(* Logix 5000 Rung export; software revision 16.04 *)

MODULES
   Local : vendor None type None code None
   MVI56E_AFC : vendor None type None code None
END_MODULES

TYPE AFCEProveProcess :   // Prove process output from processor to the module
STRUCT
   Sequencing : AFCEProveSequencing;   // Prover sequencing
   Temperature : REAL;   // Temperature for Single Probe provers. And Inlet Temperature for Dual Probe Provers.
   OutletTemperature : REAL;   // Outlet Temperature for Provers with Dual Probes.
   SwitchBarTemperature : REAL;   // Switch bar temperature
   Pressure : REAL;   // Pressure for Single Probe provers. And Inlet Pressure for Dual Probe Provers.
   OutletPressure : REAL;   // Outlet Pressure for Provers with Dual Probes.
   ProverDensity : REAL;   // Prover density
END_STRUCT
END_TYPE

TYPE AFCEMeterControl :   // Enable/Disable Meter and Streams
STRUCT
   Meter : AFCEMeterControlMeter;   // Control the Meter
   Stream : AFCEMeterControlStream;   // Control the Meter Streams
   ResetAccumulators : AFCEMeterSignals;   // Resets for meter accumulators
END_STRUCT
END_TYPE

TYPE AFCEModbusMasterDataType :   // Modbus master data type
STRUCT
   Bit : BOOL;   // bit type
   Word : BOOL;   // word type (16-bit)
   Long : BOOL;   // long integer (32-bit)
   LongRemote : BOOL;   // long integer (32-bit)
END_STRUCT
END_TYPE

TYPE AFCEProveSequencing :   // AFC prove sequencing tag for phase selection and ball positioning
STRUCT
   Phase : AFCEProvePhaseBitmap;   // AFC phase sequencing
   BallPositionReady : BOOL;   // Ball position: Ready (Udir & Bdir only; fwd leg Bdir)
   BallPositionSealed : BOOL;   // Ball position: Sealed (Udir & Bdir only; fwd leg Bdir)
   BallPositionReadyBwdLeg : BOOL;   // Ball position: Ready bwd leg (Bdir only)
   BallPositionSealedBwdLeg : BOOL;   // Ball position: Sealed bwd leg (Bdir only)
END_STRUCT
END_TYPE

TYPE AFCEMeterDifferentialLiquid :   // Differential Liquid Meter
STRUCT
   Control : AFCEMeterControl;   // Meter Control
   Status : AFCEMeterStatus;   // Meter Status
   ProcessVariables : AFCEMeterDifferentialLiquidProcess;   // Input process variables to be transferred to the module
   Alarm : AFCEMeterDifferentialLiquidAlarm;   // Meter Alarms
   Archive : AFCEMeterDifferentialLiquidArchive;   // Archive
   Profile : AFCEMeterProfile;   // Module profile (meter type/product group) transfered from the module
   Calibration : AFCEMeterDifferentialLiqCal;   // Calibration
   BackPlaneReturn : AFCEMeterDifferentialLiqBackPlaneReturn;
END_STRUCT
END_TYPE

TYPE AFCEMeterDifferentialLiquidArchiveWrite :   // Write Archive
STRUCT
   Daily : BOOL;   // Set to 1 to write daily archive
   Hourly : BOOL;   // Set to 1 to write hourly archive
END_STRUCT
END_TYPE

TYPE AFCEUtil :   // Used for internal ladder logic usage. These values must not be changed by user application.
STRUCT
   Flags : AFCEFlag;   // Wallclock update commands
   CycleCounter : INT;   // Reflects current block ID calculated by ladder to be sent to the module
   Buffer : AFCEUtilBuffer;
   Block : AFCEUtilBlock;
END_STRUCT
END_TYPE

TYPE AFCEExtended :
STRUCT
   Trigger : BOOL;
   Data : AFCEExtendedData;
END_STRUCT
END_TYPE

TYPE AFCEModbusGatewayCommand :   // Modbus Gateway Command
STRUCT
   Config : AFCEModbusGatewayConfig;   // Config data to be entered by the user.
   Trigger : BOOL;   // Trigger the Command, when cleared module has responded.
   Data : INT[200];   // Contains modbus data written to the module (write commands)
END_STRUCT
END_TYPE

TYPE AFCEMeterDifferentialLiquidArchiveFetchT :   // Fetch Archive
STRUCT
   Trigger : BOOL;   // Trigger Archive Fetch
   Age : INT;   // 0 = Current Archive
   Error : AFCEMeterArchiveFetchError;   // Archive Fetch Error
   Default : AFCEMeterDifferentialLiquidArchiveDflt;   // Default Archive
   Raw : INT[100];   // Raw Archive
END_STRUCT
END_TYPE

TYPE AFCEMeterDifferentialLiqCal :   // Processor Mediated Calibration
STRUCT
   Request : AFCEMeterDifferentialLiqCalRequest;   // Calibration Request from module
   Response : AFCEMeterCalResponse;   // Processor Response
END_STRUCT
END_TYPE

TYPE AFCEMeterStatusStream :
STRUCT
   Active : INT;   // Current Active Stream
   Enabled : AFCEMeterStatusStreamEnabled;   // Enabled Streams
   Configured : AFCEMeterStatusStreamEnabled;   // Configured Streams
   EnableAlarm : AFCEMeterStatusStreamAlarm;   // Enable Alarms
END_STRUCT
END_TYPE

TYPE AFCEProveRunResults :   // Run results of the prove. Copied from the module to the pocessor
STRUCT
   CountAttempted : INT;   // Run count attempted
   CountCompleted : INT;   // Run count completed
   CountSelected : INT;   // Run count selected
   RunsSelected : INT;   // Bit Mapped Runs selected for calculations from completed runs
   NewMeterFactor : REAL;   // New meter factor
   ChangeInMeterFactor : REAL;   // Change in meter factor
END_STRUCT
END_TYPE

TYPE AFCEModbusMasterSwap :   // Modbus master swap words/ swap bytes
STRUCT
   SwapWords : BOOL;   // Swap words
   SwapBytes : BOOL;   // Swap bytes
END_STRUCT
END_TYPE

TYPE AFCEModbusMaster :   // Modbus Master. Port 3 must be configured as modbus master through AFC Manager to use this feature.
STRUCT
   Enable : BOOL;   // Enable the modbus master funcionality
   CommandIndex : INT;   // Selects which command index will be executed
   Command : AFCEModbusMasterCommand[10];   // Each command contains a specific modbus request to be sent out of the port
END_STRUCT
END_TYPE

TYPE AFCEMeterDifferentialLiqStandardDflt :   // Differential Liquid Meter Default Standard Data
STRUCT
   Meter_Alarms : DINT;   // Meter alarms
   NR_Acc_Net_Totalizer : DINT;   // Non-resettable accumulator, net, totalizer (m3)
   NR_Acc_Net_Residue : REAL;   // Non-resettable accumulator, net, residue (m3)
   FlowRate_Net : REAL;   // Flow rate, net (m3/h)
   NR_Acc_Gross_Totalizer : DINT;   // Non-resettable accumulator, gross, totalizer (m3)
   NR_Acc_GrossStandard_Totalizer : DINT;   // Non-resettable accumulator, gross standard, totalizer (m3)
   NR_Acc_Mass_Totalizer : DINT;   // Non-resettable accumulator, mass, totalizer (kg)
END_STRUCT
END_TYPE

TYPE AFCEFlag :   // Flags contains status information updated by ladder and also trigger bits for clock update
STRUCT
   AFCStopped : BOOL;   // Indicates that the module has sent a new input block to be processed by ladder - UPDATED BY LADDER
   AFCInputSequenceNum : INT;   // Meter number (0 -15) associated to blocks 1-16. Used to update "Profile" (meter type and product group.) UPDATED BY LADDER
END_STRUCT
END_TYPE

TYPE AFCEModbusPassThruBitData :   // AFC Modbus Pass-thru Bit Data
STRUCT
   Data : BOOL[2016];   // Contains received data for bit commands
END_STRUCT
END_TYPE

TYPE AFCEUtilBlockInterrupt :
STRUCT
   Now : BOOL;
   ModbusGateway : DINT;
   EnableDisable : BOOL;
   Analysis : DINT;
END_STRUCT
END_TYPE

TYPE AFCEFirmwareVersion :
STRUCT
   Major : SINT;   // Major Version number
   Minor : SINT;   // Minor Version number
   Revision : INT;   // Revision
END_STRUCT
END_TYPE

TYPE AFCEModbusGateway :   // Modbus Gateway
STRUCT
   Command : AFCEModbusGatewayCommand[10];   // Modbus gateway commands - contains setup and modbus data
END_STRUCT
END_TYPE

TYPE AFCEMeterDifferentialLiquidArchive :   // Different Liquid Archive
STRUCT
   Write : AFCEMeterDifferentialLiquidArchiveWrite;
   Fetch : AFCEMeterDifferentialLiquidArchiveFetch;
END_STRUCT
END_TYPE

TYPE AFCEMeterCalRequestActionType :
STRUCT
   ZeroShift : BOOL;   // Zero Shift
   SetZero : BOOL;   // Set Zero
   SetSpan : BOOL;   // Set Span
   SetMid1 : BOOL;   // Set Mid 1
   SetMid2 : BOOL;   // Set Mid 2
   SetMid3 : BOOL;   // Set Mid 3
END_STRUCT
END_TYPE

TYPE AFCEUtilBuffer :   // Buffer
STRUCT
   Input : INT[250];   // Input buffer contains the complete block to be copied from the module
   Output : INT[248];   // Output buffer contains data the complete block to be copied to the module
   Process : INT[240];
   ArchiveDay : INT[98];
   ArchiveHour : INT[98];
   Prove : INT[26];
   Analysis : INT[198];
   MeterEnableDisable : INT[4];
   StreamEnable : INT[48];
   StreamDisable : INT[48];
   StreamSelect : INT[32];
   MeterSignals : INT[32];
   Calibration : INT[36];
END_STRUCT
END_TYPE

TYPE AFCEUtilBlock :
STRUCT
   ProcessInput : INT;
   InterruptPending : AFCEUtilBlockInterrupt;
   InterruptComplete : AFCEUtilBlockInterrupt;
   NonInterruptPending : AFCEUtilBlockNonInterrupt;
   NonInterruptComplete : AFCEUtilBlockNonInterrupt;
END_STRUCT
END_TYPE

TYPE AFCEMeterSignals :   // Meter trigger accumulator and archive resets
STRUCT
   ResetAccumulator1 : BOOL;   // Set to 1 to reset resettable accumulator 1
   ResetAccumulator2 : BOOL;   // Set to 1 to reset resettable accumulator 2
   ResetAccumulator3 : BOOL;   // Set to 1 to reset resettable accumulator 3
   ResetAccumulator4 : BOOL;   // Set to 1 to reset resettable accumulator 4
END_STRUCT
END_TYPE

TYPE AFCEProve :   // Prove
STRUCT
   Process : AFCEProveProcess;   // Process Variables
   Signals : AFCEProveSignals;   // AFC Prove Signals (triggers the proving update)
   Config : AFCEProveConfig;   // AFC Prove Control (configuration settings)
   PulseCounts : AFCEProvePulseCount;   // Pulse counts to be updated at the end of the run/pass
   ConfigInput : AFCEProveInputConfig;   // AFC prover input configuration
   Status : AFCEProveStatus;   // AFC prover status
   ErrorCode : INT;   // Prove error code
   ProveControlsEcho : INT;   // AFC module Echos the state of the Prove Controls
   RequestedMeterEcho : INT;   // AFC module Echos the Meter number requested
   RequestedCurvePointEcho : INT;   // AFC module Echos the requested Curve Point
   RunResults : AFCEProveRunResults;   // Prove and run results
   ProveEnabled : BOOL;   // ON if prove is enabled. This flag is coped from inputbuffer[247]
END_STRUCT
END_TYPE

TYPE AFCEMeterControlStream :
STRUCT
   Selected : SINT;   // Stream to Enable or Disable and/or make active.
   EnableSelected : BOOL;   // Enable the Selected Stream
   DisableSelected : BOOL;   // Disable the Selected Stream
   SetSelectedToActive : BOOL;   // Set Selected to Active Stream
END_STRUCT
END_TYPE

TYPE AFCEProveConfig :   // Controls (configuration settings) associated to the prover
STRUCT
   Enable : AFCEProveConfigEnable;   // Controls at enable
   Accept : AFCEProveConfigAccept;   // Controls at accept
END_STRUCT
END_TYPE

TYPE AFCEWallclock :
STRUCT
   GetAFCTime : BOOL;   // Get current AFC Time
   SetAFCTimeFromPLCTime : BOOL;   // Set AFC time from PLC time. Updates current AFC time
   EnableLocalDateTime : BOOL;   // Enable Local Date Time.
   AFCTime : AFCETime;   // Coordinated Universal Time. Updated by either getting or setting AFC time.
END_STRUCT
END_TYPE

TYPE AFCEMeterCalRequestActionValue :
STRUCT
   ZeroShift : AFCEMeterCalRequestValue;   // Zero Shift
   SetZero : AFCEMeterCalRequestValue;   // Set Zero
   SetSpan : AFCEMeterCalRequestValue;   // Set Span
   SetMid1 : AFCEMeterCalRequestValue;   // Set Mid 1
   SetMid2 : AFCEMeterCalRequestValue;   // Set Mid 2
   SetMid3 : AFCEMeterCalRequestValue;   // Set Mid 3
END_STRUCT
END_TYPE

TYPE AFCEMeterStatus :   // Status
STRUCT
   Meter : AFCEMeterStatusMeter;   // Meter Status
   Stream : AFCEMeterStatusStream;   // Stream Status
END_STRUCT
END_TYPE

TYPE AFCEMeterDifferentialLiquidAlarmControl :   // Differential Liquid Process Alarms
STRUCT
   DifferentialPressure : AFCEMeterProcessAlarm;   // Differential Pressure Alarms
   FlowRate : AFCEMeterProcessAlarm;   // Flow Rate Alarms
   Temperature : AFCEMeterProcessAlarm;   // Temperature Alarms
   Pressure : AFCEMeterProcessAlarm;   // Pressure Alarms
   Density : AFCEMeterProcessAlarm;   // Density Alarms
   WaterPercent : AFCEMeterProcessAlarm;   // Differential Pressure Alarms
END_STRUCT
END_TYPE

TYPE AFCEModbusMasterConfig :   // Modbus master command settings
STRUCT
   Enable : BOOL;   // Set to 1 to enable command (0=disable)
   FunctionType : BOOL;   // Set to 1 to select write command (0=read command)
   RegisterBank : BOOL;   // Set to 1 to select input register (0=holding register)
   DataType : AFCEModbusMasterDataType;   // Select data type format
   SwapOption : AFCEModbusMasterSwap;   // Select byte and word swap (1 = swap, 0 = no swap)
   TypeSwap : INT;   // This value is calculated by ladder logic and must not be modified by user
   SlaveAddress : INT;   // Modbus slave address of remote device
   ModbusAddress : INT;   // Modbus data address on remote slave
   ElementCount : INT;   // Number of data elements (125 words)
   TransactionID : INT;   // Transaction ID. This value is returned to the ReturnedTransaction ID when the response has been received.
END_STRUCT
END_TYPE

TYPE AFCEMeterStatusStreamEnabled :   // Stream Status 1 = Enabled
STRUCT
   Stream1 : BOOL;
   Stream2 : BOOL;
   Stream3 : BOOL;
   Stream4 : BOOL;
   Stream5 : BOOL;
   Stream6 : BOOL;
   Stream7 : BOOL;
   Stream8 : BOOL;
   Stream9 : BOOL;
   Stream10 : BOOL;
   Stream11 : BOOL;
   Stream12 : BOOL;
   Stream13 : BOOL;
   Stream14 : BOOL;
   Stream15 : BOOL;
   Stream16 : BOOL;
END_STRUCT
END_TYPE

TYPE AFCEMeterArchiveFetchError :
STRUCT
   ArchiveSelectionInvalid : BOOL;   // Archive File Selection Invalid
   AgeOutsideSize : BOOL;   // Age Outside Configured File Size
   ArchiveNeverWritten : BOOL;   // Age OK but Archive Record Never Written (new or reconfigured meter)
   Reserverd1 : BOOL;
   Reserverd2 : BOOL;
   Reserverd3 : BOOL;
   Reserverd4 : BOOL;
   Reserverd5 : BOOL;
   Reserverd6 : BOOL;
   Reserverd7 : BOOL;
   Reserverd8 : BOOL;
   Reserverd9 : BOOL;
   Reserverd10 : BOOL;
   Reserverd11 : BOOL;
   Reserverd12 : BOOL;
   Reserverd13 : BOOL;
END_STRUCT
END_TYPE

TYPE AFCESiteStatus :   // Site status bits - contains general information about the module - not meter specific
STRUCT
   AFCActive : BOOL;   // AFC active
   ChecksumAlarms : BOOL;   // Checkum alarm active
   Reserved2 : BOOL;
   Reserved3 : BOOL;
   PLCHalted : BOOL;   // PLC in program mode or missing
   CfgChanged : BOOL;   // Configuration changed
   Powerup : BOOL;   // Module powered up
   ColdStart : BOOL;   // Module performed cold start (BBRAM initialized)
   ModbusMasterPending : BOOL;   // Modbus Master Poll Pending
   ModbusMasterComplete : BOOL;   // Modbus Master Poll Complete
   ModbusPassThruPending : BOOL;   // Modbus Pass-thru Input Pending
   CalibrationRequest : BOOL;   // Calibration request from module
   ProverEnabled : BOOL;   // Prover Enabled
   Reserved13 : BOOL;
   Reserved14 : BOOL;
   Reserved15 : BOOL;
END_STRUCT
END_TYPE

TYPE AFCEModuleDef :   // Main user defined data type
STRUCT
   ModbusGateway : AFCEModbusGateway;   // Reads and write data between processor and module modbus table
   ModbusMaster : AFCEModbusMaster;   // Setup modbus master commands to be sent to remote slaves (through Port 3)
   ModbusPassThru : AFCEModbusPassThru;   // Modbus pass-thru data
   SiteStatus : AFCESiteStatus;   // Site status
   MeterAlarms : AFCESiteAlarms;   // Meter Alarms
   Prove : AFCEProve;   // Prover
   Wallclock : AFCEWallclock;   // Set clock and get clock information
   Firmware : AFCEFirmwareVersion;   // Firmware information
   Util : AFCEUtil;   // Used by ladder logic
END_STRUCT
END_TYPE

TYPE AFCEModbusGatewayConfig :   // Modbus Ggateway Configuration
STRUCT
   Enable : BOOL;   // Set to 1 to enable modbus gateway command (0=disable)
   StartRegister : DINT;   // Start modbus address
   RegisterCount : INT;   // Word count (200 max)
   FunctionType : BOOL;   // 0 = read command, 1 = write command
   RegisterType : BOOL;   // 0 = holding register, 1 = input register
   SlaveType : BOOL;   // 0 = primary slave, 1 = virtual slave
END_STRUCT
END_TYPE

TYPE AFCEMeterDifferentialLiqCalRequest :
STRUCT
   ProcessVariable : AFCEMeterDifferentialLiqCalRequestProces;   // Process Variable
   ActionType : AFCEMeterCalRequestActionType;   // Action Type
   Value : AFCEMeterCalRequestActionValue;   // Value
   Count : DINT;   // Number of calibration requests
END_STRUCT
END_TYPE

TYPE AFCEMeterCalRequestValue :
STRUCT
   Applied : REAL;   // Applied
   Measured : REAL;   // Measured
END_STRUCT
END_TYPE

TYPE AFCEUtilBlockNonInterrupt :
STRUCT
   Now : BOOL;
   ModbusMasterCommand : BOOL;
   ModbusMasterResponse : BOOL;
   Archive : DINT;
   Prover : BOOL;
   PassThru : BOOL;
   Calibration : BOOL;
END_STRUCT
END_TYPE

TYPE AFCEProveConfigAccept :   // Prove controls at accept. If auto-accept is selected must be available at enable
STRUCT
   RequestedInterpolationPoint : INT;   // Requested interpolation point (0 nearest)
   ApplyMFChangeAllStreams : BOOL;   // Apply change in meter factor to all streams
   ApplyMFChangeCurve : BOOL;   // Apply change in meter factor to all curve points
   ApplyNewMF : BOOL;   // CApply new meter factor
END_STRUCT
END_TYPE

TYPE AFCEProvePhaseBitmap :   // AFC prove phase bitmap
STRUCT
   NotSelected : BOOL;   // Not selected
   Active : BOOL;   // Active, not counting
   CountingPast1stSwitch : BOOL;   // Counting past 1st switch for Udir and forward leg for Bdir)
   Past2ndSwitchFwdLeg : BOOL;   // Past 2nd switch forward leg (bidirectional only)
   Past1stSwithRetLeg : BOOL;   // Past 1st switch return leg (bidirectional only)
   RunComplete : BOOL;   // Run complete. past 2nd switch.
END_STRUCT
END_TYPE

TYPE AFCETime :   // AFC time format used for wallclock update.
STRUCT
   Year : DINT;   // Year
   Month : DINT;   // Month
   Day : DINT;   // Day
   Hour : DINT;   // Hour
   Minute : DINT;   // Minute
   second : DINT;   // Seconds
END_STRUCT
END_TYPE

TYPE AFCEMeterDifferentialLiquidArchiveFetch :
STRUCT
   Daily : AFCEMeterDifferentialLiquidArchiveFetchT;
   Hourly : AFCEMeterDifferentialLiquidArchiveFetchT;
END_STRUCT
END_TYPE

TYPE AFCEProveSignals :   // Contains the proving signals that will trigger specific tasks from the module
STRUCT
   EnableProve : BOOL;   // Enables the prove
   AcceptProve : BOOL;   // Accepts the prove
   RejectProve : BOOL;   // Reject the prove
   RunStart : BOOL;   // Starts the run
   RunComplete : BOOL;   // Flags that the run is complete
   RunCancel : BOOL;   // Cancels the run
   RunDelete : BOOL;   // Deletes the run
   PassComplete : BOOL;   // Flag that the pass is complete
   PauseProve : BOOL;   // Pauses the Proving Process
   AbortProve : BOOL;   // Aborts the prove
END_STRUCT
END_TYPE

TYPE AFCEMeterProfile :   // Meter configuration profile
STRUCT
   MeterType : BOOL;   // 0=Differential, 1=Linear
   ProductGroup : BOOL;   // 0=Gas, 1=Liquid
   PrimaryInput : BOOL;   // For differential, 0=Differential Pressure 1=Flow Rate. For Linear, 0=Pulse Count 1=Pulse Frequency
   AOIMismatch : BOOL;   // AOI Meter type does not match module for meter number
END_STRUCT
END_TYPE

TYPE AFCEMeterStatusStreamAlarm :   // Stream Alarms
STRUCT
   StreamOutOfRange : BOOL;   // Requested Stream Number Out of Range
   StreamNotConfigured : BOOL;   // Requested Stream not Configured
   StreamNotEnabled : BOOL;   // Requested Stream not Enabled
   EventLogFull : BOOL;   // Event Log Full, Action not Performed
END_STRUCT
END_TYPE

TYPE AFCEModbusPassThru :   // AFC Modbus Pass-thru
STRUCT
   Enable : BOOL;   // Set to 1 to enable pass-thru functionality (requires AFC Manager setting)
   MessagePresent : BOOL;   // Message present in the response block
   GetMessage : BOOL;   // Get the pass-thru message. When the bit is cleared the message has been transferred to the PLC.
   FunctionBitWrite : BOOL;   // Function bit write
   OverflowError : BOOL;   // Overflow error flag
   ModbusAddress : INT;   // Destination modbus address
   RegisterCount : INT;   // Number of elements associated to command
   ReadDataWord : INT[125];   // Contains received data for word commands
   ReadDataBit : AFCEModbusPassThruBitData;   // Contains received data for bit commands
END_STRUCT
END_TYPE

TYPE AFCEProveInputConfig :   // Prove input block results - prover configuration
STRUCT
   Type : INT;   // Prover type
   Options : INT;   // Prover options
   RunsPerProveTotal : INT;   // Total runs per prove
   RunsPerProveSelected : INT;   // Selected runs per prove
   MaxRunsBeforeAbort : INT;   // Max total runs before abort
   ShortPassesPerRun : INT;   // Short passes per run if bidir = 2 , else 0
END_STRUCT
END_TYPE

TYPE AFCEProveStatus :   // Status of the prove (returned from the module to the processor)
STRUCT
   ProveAccepted : BOOL;   // Prove was accepted
   MeterFactorApplied : BOOL;   // Meter factor was applied
   MFAppliedToCurve : BOOL;   // Meter factor was applied to all points in the curve
   MFAppliedToStreams : BOOL;   // Meter factor was applied to all streams
   ProveRejectedByCommand : BOOL;   // Prove was rejected by command
   ProveRejectedNoRuns : BOOL;   // Prove was rejected - empty prove (no runs)
   ProveRejectedDivideBy0 : BOOL;   // Prove was rejected - divide by 0
   ProveEnabled : BOOL;   // Prove is enabled
   ProvingRunInProgress : BOOL;   // Proving run is in progress
   ProveRejectedAbort : BOOL;   // Prove rejected: abort
   ProvePaused : BOOL;   // Prove is paused
   RunCancelled : BOOL;   // Run Is cancelled
   RunTimedOut : BOOL;   // Run timed out
END_STRUCT
END_TYPE

TYPE AFCEMeterProcessAlarm :   // Process Alarms
STRUCT
   SetGeneralFail : BOOL;   // Set to indicate General Failure of the Transmitter
   StaleData : BOOL;   // Clear to Indicate new process input data
   SetLowThreshold : BOOL;   // Set to indicate Lower Range Limit Exceeded
   SetHighThreshold : BOOL;   // Set to indicate Upper Range Limit Exceeded
   SetAutoClearStaleData : BOOL;   // Set to automatically clear stale data
END_STRUCT
END_TYPE

TYPE AFCEProveConfigEnable :   // Prove controls at enable
STRUCT
   MeterNumber : INT;   // Meter number requested (1-16)
   AutoAcceptProve : BOOL;   // Auto-accept the prove
   AutoContinueProve : BOOL;   // Auto-continue the prove
END_STRUCT
END_TYPE

TYPE AFCEMeterStatusMeter :   // Meter Status
STRUCT
   Enabled : BOOL;   // Meter Enable Status, 1=enabled
   EnableAlarm : BOOL;   // If set either: 1. The meter is not configured. 2. The event log is full, the action was not performed.
END_STRUCT
END_TYPE

TYPE AFCEMeterDifferentialLiquidAlarm :
STRUCT
   Control : AFCEMeterDifferentialLiquidAlarmControl;   // Alarm Control
END_STRUCT
END_TYPE

TYPE AFCEMeterControlMeter :   // Enable and Disable Meter
STRUCT
   Enable : BOOL;   // Enable the Meter
   Disable : BOOL;   // Disable the Meter
END_STRUCT
END_TYPE

TYPE AFCEModbusMasterCommand :   // Modbus Master Command
STRUCT
   Config : AFCEModbusMasterConfig;   // Modbus Master Configuration
   ErrorCode : INT;   // Error Code associated to Modbus Master Command
   Pending : BOOL;   // Pending Modbus Master Command - waiting for Modbus Response
   ReturnedTransactionID : DINT;   // Changes to Config.TransactionID value when response has returned.
   Data : INT[100];   // Read or Write Data
END_STRUCT
END_TYPE

TYPE AFCEMeterDifferentialLiqCalRequestProces :
STRUCT
   DifferentialPressure : BOOL;   // Differential Pressure
   Temperature : BOOL;   // Temperature
   Pressure : BOOL;   // Pressure
   Density : BOOL;   // Density
   WaterContent : BOOL;   // Water Content
END_STRUCT
END_TYPE

TYPE AFCEMeterDifferentialLiquidProcess :   // Differential Liquid Process Variables
STRUCT
   DifferentialPressure : REAL;   // Differential pressure if Primary Input = Differential pressure
   FlowRate : REAL;   // Flow rate if Primary Input = Flow rate
   Temperature : REAL;   // Temperature
   Pressure : REAL;   // Static Pressure
   Density : REAL;   // Density
   WaterPercent : REAL;   // Water %
END_STRUCT
END_TYPE

TYPE AFCEProvePulseCount :   // Values to be supplied at the end of the pass/run
STRUCT
   Meter : DINT;   // Meter pulse count
   MasterMeter : DINT;   // Master meter pulse count
END_STRUCT
END_TYPE

TYPE AFCEMeterCalResponse :
STRUCT
   Trigger : BOOL;   // Send Error Code and Values to module to be recorded
   ErrorCode : SINT;   // Error Code to send. 0-4 allowed. 0=No error. 1-4=User defined.
   Value : AFCEMeterCalRequestValue;   // Value to Send
   Count : DINT;   // Number of calibration responses
END_STRUCT
END_TYPE

TYPE AFCEExtendedData :
STRUCT
   Raw : INT[64];
END_STRUCT
END_TYPE

TYPE AFCEMeterDifferentialLiquidArchiveDflt :   // Default Configuration
STRUCT
   ClosingTimestamp : DINT;
   CumulativeActiveStreams : INT;
   CurrentActiveStream : SINT;
   MeterStatus : SINT;
   FlowingPeriod : DINT;
   PeriodDuration : DINT;
   AccumulatorTotalizer : DINT;
   AccumulatorResidue : REAL;
   MeterAlarms : DINT;
   PrimaryInput : REAL;   // Either Differential Pressure or Flow Rate
   Temperature : REAL;
   Pressure : REAL;
   Density : REAL;
   WaterContent : REAL;
   ReferenceDensity : REAL;
   Ctpl : REAL;
   AGA3DensityExtension : REAL;
   AGA3CoefficientDischarge : REAL;
   Available01 : INT;
   Available02 : INT;
   Cprime : REAL;
   MassNRAccumulatorCurrent : REAL;   // Non-resettable
   MassNRAccumulatorOpening : REAL;   // Non-resettable
   Available03 : INT;
   Available04 : INT;
   Available05 : INT;
   Available06 : INT;
   NetNRAccumulatorCurrent : REAL;   // Non-resettable
   NetNRAccumulatorOpening : REAL;   // Non-resettable
   GrossNRAccumulatorCurrent : REAL;   // Non-resettable
   GrossNRAccumulatorOpening : REAL;   // Non-resettable
   GrossStandardNRAccumulatorOpening : REAL;   // Non-resettable
   GrossStandardNRAccumulatorCurrent : REAL;   // Non-resettable
   WaterNRAccumulatorCurrent : REAL;   // Non-resettable
   WaterNRAccumulatorOpening : REAL;   // Non-resettable
   API2540VaporPressureAbs : REAL;
   Available07 : INT;
   Available08 : INT;
   UserSpecifiedFlowAveraged1 : REAL;
   UserSpecifiedFlowAveraged2 : REAL;
   UserSpecifiedFlowAveraged3 : REAL;
END_STRUCT
END_TYPE

TYPE AFCEMeterDifferentialLiqBackPlaneReturn :   // Differential Liquid Meter
STRUCT
   StandardDefault : AFCEMeterDifferentialLiqStandardDflt;
   StandardRaw : INT[14];
   Extended : AFCEExtended;
END_STRUCT
END_TYPE

TYPE AFCESiteAlarms :   // Indicates if a meter has any alarms
STRUCT
   Meter1 : BOOL;   // Meter in alarm
   Meter2 : BOOL;   // Meter in alarm
   Meter3 : BOOL;   // Meter in alarm
   Meter4 : BOOL;   // Meter in alarm
   Meter5 : BOOL;   // Meter in alarm
   Meter6 : BOOL;   // Meter in alarm
   Meter7 : BOOL;   // Meter in alarm
   Meter8 : BOOL;   // Meter in alarm
   Meter9 : BOOL;   // Meter in alarm
   Meter10 : BOOL;   // Meter in alarm
   Meter11 : BOOL;   // Meter in alarm
   Meter12 : BOOL;   // Meter in alarm
   Meter13 : BOOL;   // Meter in alarm
   Meter14 : BOOL;   // Meter in alarm
   Meter15 : BOOL;   // Meter in alarm
   Meter16 : BOOL;   // Meter in alarm
END_STRUCT
END_TYPE

ADD_ON_INSTRUCTION AOI56EAFCMeterDifferentialLiquid   (* revision 1.8, vendor ProSoft Technology Inc., ExecutePrescan *)
// Add-On instruction for the MVI56E-AFC.
// Differential Liquid Meter
// Revision note:
// Corrected/Reverted ProcessInputBlockID Tag Data Type from INT to DINT.
// Help:
// Compatible with version 4.03 of MVI56E-AFC firmware or higher.
// v1.2: Remove Calculation Results. Add Backplane Return. Add Stale Data
// v1.3: Added Flow Rate Process Input and Flow Rate Alarm Controller Tags for Flow Rate Devices (and not just for Differential Pressure)
// v1.4: Addition of default process input backplane return data mapping.
// v1.5: Made correlation changes between the Module Archive Default UDTs and the AOI Archive Default
// UDTs
// v1.6: Made changes to the Flow Rate Primary Input Block ID Insertion in Rung 8 (Removed +1), Modified ProcessInputBlockID Tag Data Type from DINT to INT, and modified ModbusGatewayConfig UDT StartRegister Tag Data Type from INT to DINT.
// v1.7: Updated Tags names AFCMeterXXYYYYYY.BackPlaneReturn.ProcessInputs to
// AFCMeterXXYYYYYY.BackPlaneReturn.Standard and
// AFCMeterXXYYYYYY.BackPlaneReturn.ComponentAnalysis
//  to AFCMeterXXYYYYYY.BackPlaneReturn.Extended.
// v1.8:  Corrected/Reverted ProcessInputBlockID Tag Data Type from INT to DINT.
VAR_IN_OUT
   ConnectionInput : INT[250]; {required}
   AFC : AFCEModuleDef; {required}
   AFCMeter : AFCEMeterDifferentialLiquid; {required}
END_VAR
VAR_INPUT
   MeterNumber : SINT; {required}   // Meter Number Set to a number between 1 and 16
END_VAR
VAR
   StreamSelectedShift : DINT;
   StreamSelectBuffer : INT;
   EnabledStatusBuffer : INT;
   StreamSelectBlockID : DINT;
   StreamNumberShift : DINT;
   StreamErrorBuffer : DINT;
   StreamEnableBlockID : DINT;
   StreamEnableBitPosition : DINT;
   StreamDisableBlockID : DINT;
   ProfileBuffer : SINT[2];
   ProcessInputBlockID : DINT;
   CalibrationHandleBuffer : INT;
   AnalysisGroupBitPosition : INT;
   ProcessAlarmShifter : DINT;
   ProcessAlarmHolder : DINT;
   ProcessAlarmBuffer : DINT;
   MeterSignaltBlockID : DINT;
   MeterNumberShift : DINT;
   MeterNumberBitPostition : DINT;
   Inputbuffer : INT[250];
   CalibrationMeterNumberBuffer : DINT;
   CalibrationMediationPending : BOOL;
   CalibrationInputScalingIndex : DINT;
   AnalysisErrorBuffer : INT;
   ArchiveStream : DINT;
   ArchiveMeterStatusRaw : DINT;
   ArchiveMeterStatusActiveStream : DINT;
   ArchiveCompleteBitCheck : DINT;
   ArchiveBlockID : DINT;
   AnalysisGroupShift : DINT;
   AnalysisCompleteBitCheck : DINT;
   AnalysisBufferOffset : DINT;
   AFCStopped : BOOL;
   AFCInputDataAvailable : BOOL;
   AnalysisBlockID : DINT;
END_VAR

ROUTINE Logic   (* ladder *)
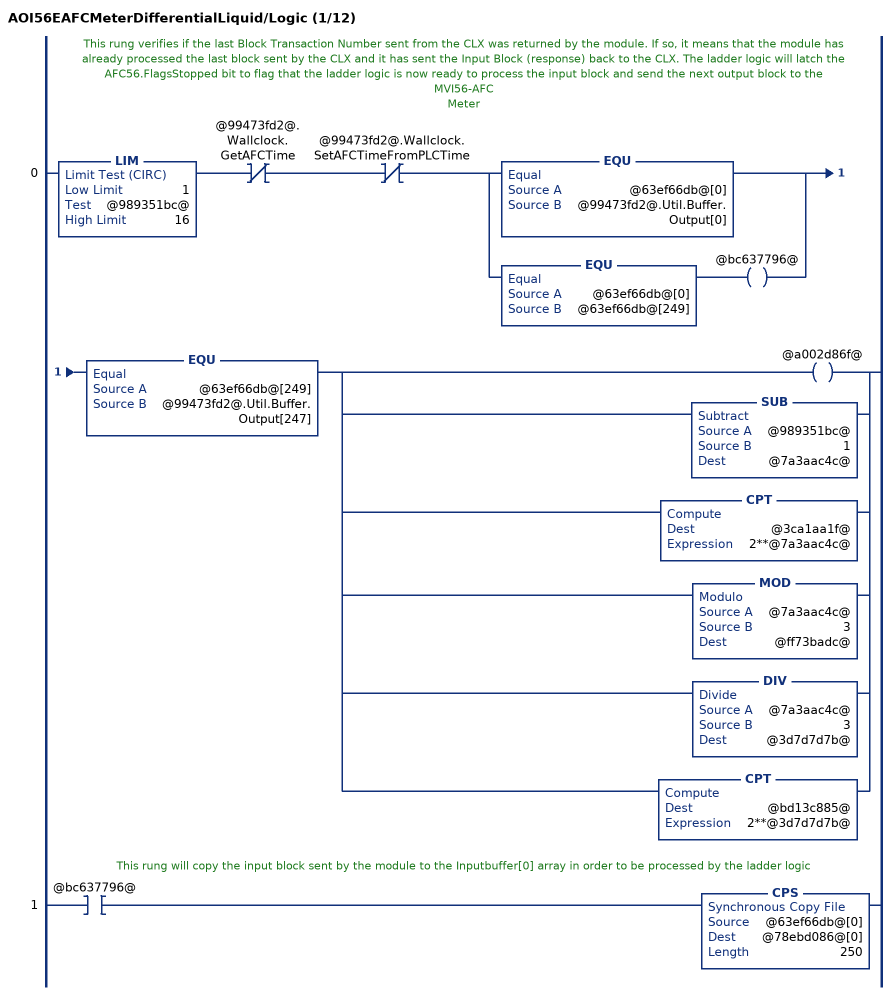
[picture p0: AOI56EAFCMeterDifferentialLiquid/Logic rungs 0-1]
   // This rung verifies if the last Block Transaction Number sent from the CLX was returned by the module. If so, it means that the module has already processed the last block sent by the CLX and it has sent the Input Block (response) back to the CLX. The ladder logic will latch the AFC56.FlagsStopped bit to flag that the ladder logic is now ready to process the input block and send the next output block to the MVI56-AFC
   // Meter
   0: LIM(1,@989351bc@,16)XIO(@99473fd2@.Wallclock.GetAFCTime)XIO(@99473fd2@.Wallclock.SetAFCTimeFromPLCTime)[EQU(@63ef66db@[0],@99473fd2@.Util.Buffer.Output[0]) ,EQU(@63ef66db@[0],@63ef66db@[249]) OTE(@bc637796@) ]EQU(@63ef66db@[249],@99473fd2@.Util.Buffer.Output[247])[OTE(@a002d86f@) ,SUB(@989351bc@,1,@7a3aac4c@) ,CPT(@3ca1aa1f@,2**@7a3aac4c@) ,MOD(@7a3aac4c@,3,@ff73badc@) ,DIV(@7a3aac4c@,3,@3d7d7d7b@) ,CPT(@bd13c885@,2**@3d7d7d7b@) ];
   // This rung will copy the input block sent by the module to the Inputbuffer[0] array in order to be processed by the ladder logic
   1: XIC(@bc637796@)CPS(@63ef66db@[0],@78ebd086@[0],250);
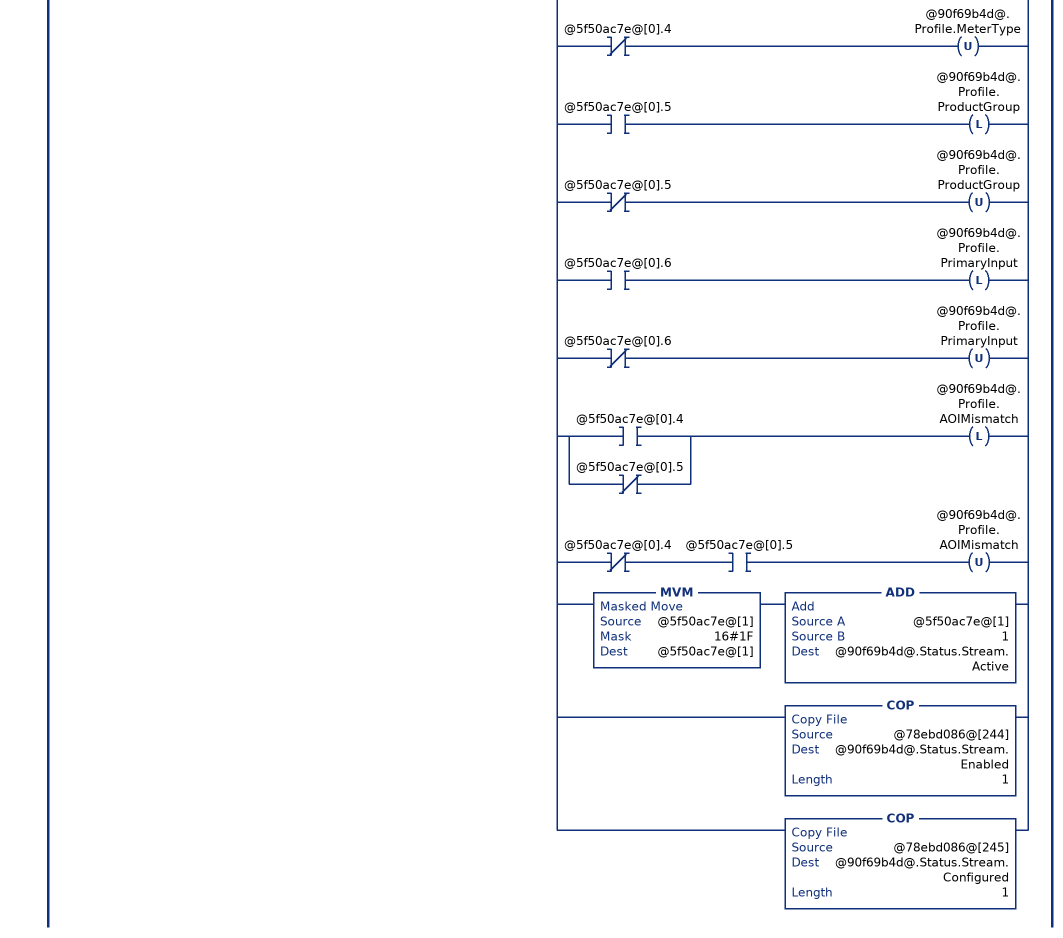
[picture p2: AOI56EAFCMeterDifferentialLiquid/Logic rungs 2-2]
   // Read process input backplane return and
   // meter profile (when block ID matches meter number).
   2: XIC(@bc637796@)LIM(1,@78ebd086@[0],16)[COP(@78ebd086@[3+@7a3aac4c@*15],@90f69b4d@.BackPlaneReturn.StandardRaw[0],14) ,COP(@90f69b4d@.BackPlaneReturn.StandardRaw[0],@90f69b4d@.BackPlaneReturn.StandardDefault,1) ,COP(@78ebd086@[247],@99473fd2@.SiteStatus,1) ,COP(@78ebd086@[248],@99473fd2@.MeterAlarms,1) ,EQU(@78ebd086@[0],@989351bc@) [COP(@78ebd086@[243],@5f50ac7e@[0],2) ,[XIC(@5f50ac7e@[0].0) OTL(@90f69b4d@.Status.Meter.EnableAlarm) ,XIO(@5f50ac7e@[0].0) OTU(@90f69b4d@.Status.Meter.EnableAlarm) ] ,[XIC(@5f50ac7e@[0].1) OTL(@90f69b4d@.Status.Meter.Enabled) ,XIO(@5f50ac7e@[0].1) OTU(@90f69b4d@.Status.Meter.Enabled) ] ,[[XIC(@5f50ac7e@[0].4) OTL(@90f69b4d@.Profile.MeterType) ,XIO(@5f50ac7e@[0].4) OTU(@90f69b4d@.Profile.MeterType) ] ,[XIC(@5f50ac7e@[0].5) OTL(@90f69b4d@.Profile.ProductGroup) ,XIO(@5f50ac7e@[0].5) OTU(@90f69b4d@.Profile.ProductGroup) ] ,[XIC(@5f50ac7e@[0].6) OTL(@90f69b4d@.Profile.PrimaryInput) ,XIO(@5f50ac7e@[0].6) OTU(@90f69b4d@.Profile.PrimaryInput) ] ] ,[[XIC(@5f50ac7e@[0].4) ,XIO(@5f50ac7e@[0].5) ] OTL(@90f69b4d@.Profile.AOIMismatch) ,XIO(@5f50ac7e@[0].4) XIC(@5f50ac7e@[0].5) OTU(@90f69b4d@.Profile.AOIMismatch) ] ,MVM(@5f50ac7e@[1],16#1F,@5f50ac7e@[1]) ADD(@5f50ac7e@[1],1,@90f69b4d@.Status.Stream.Active) ,COP(@78ebd086@[244],@90f69b4d@.Status.Stream.Enabled,1) ,COP(@78ebd086@[245],@90f69b4d@.Status.Stream.Configured,1) ] ];
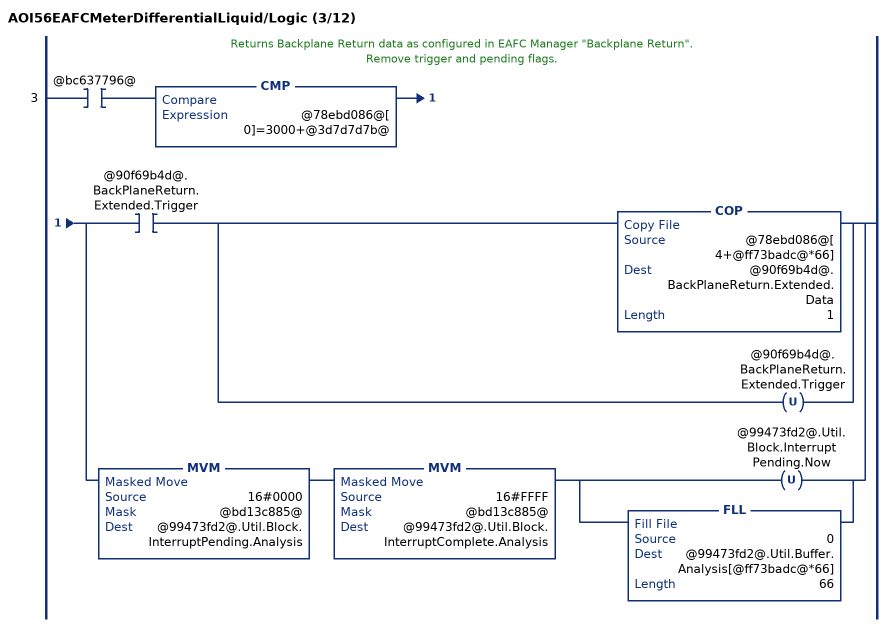
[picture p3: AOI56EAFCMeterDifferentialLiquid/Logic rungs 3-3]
   // Returns Backplane Return data as configured in EAFC Manager "Backplane Return".
   // Remove trigger and pending flags.
   3: XIC(@bc637796@)CMP(@78ebd086@[0]=3000+@3d7d7d7b@)[XIC(@90f69b4d@.BackPlaneReturn.Extended.Trigger) [COP(@78ebd086@[4+@ff73badc@*66],@90f69b4d@.BackPlaneReturn.Extended.Data,1) ,OTU(@90f69b4d@.BackPlaneReturn.Extended.Trigger) ] ,MVM(16#0000,@bd13c885@,@99473fd2@.Util.Block.InterruptPending.Analysis) MVM(16#FFFF,@bd13c885@,@99473fd2@.Util.Block.InterruptComplete.Analysis) [OTU(@99473fd2@.Util.Block.InterruptPending.Now) ,FLL(0,@99473fd2@.Util.Buffer.Analysis[@ff73badc@*66],66) ] ];
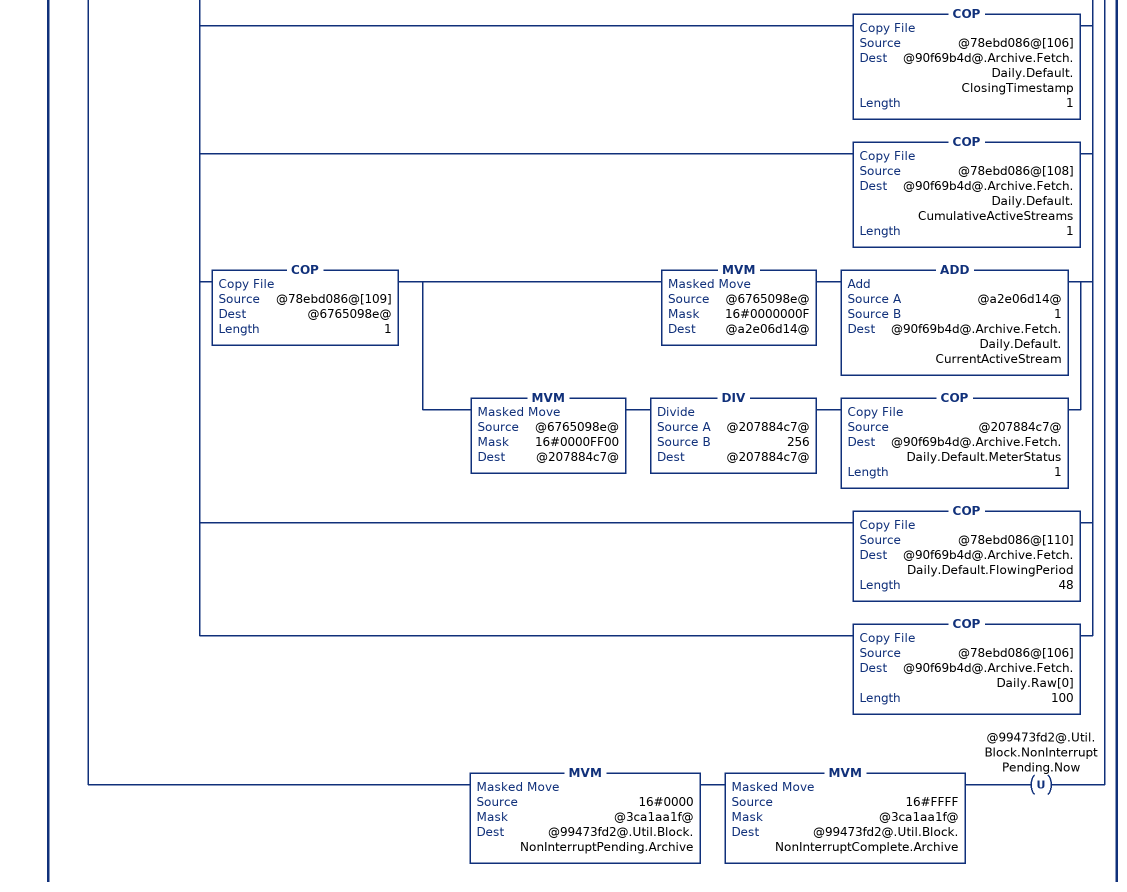
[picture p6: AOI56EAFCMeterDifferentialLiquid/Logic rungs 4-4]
   // Archive Fetch to default and raw UDT's.
   // Get archive alarms.
   // Remove trigger and pending flags.
   4: XIC(@bc637796@)CMP(@78ebd086@[0]=6000+@7a3aac4c@)[XIC(@90f69b4d@.Archive.Fetch.Hourly.Trigger) [OTU(@90f69b4d@.Archive.Fetch.Hourly.Trigger) ,[[XIC(@78ebd086@[3].0) OTL(@90f69b4d@.Archive.Fetch.Hourly.Error.ArchiveSelectionInvalid) ,XIO(@78ebd086@[3].0) OTU(@90f69b4d@.Archive.Fetch.Hourly.Error.ArchiveSelectionInvalid) ] ,[XIC(@78ebd086@[3].1) OTL(@90f69b4d@.Archive.Fetch.Hourly.Error.AgeOutsideSize) ,XIO(@78ebd086@[3].1) OTU(@90f69b4d@.Archive.Fetch.Hourly.Error.AgeOutsideSize) ] ,[XIC(@78ebd086@[3].2) OTL(@90f69b4d@.Archive.Fetch.Hourly.Error.ArchiveNeverWritten) ,XIO(@78ebd086@[3].2) OTU(@90f69b4d@.Archive.Fetch.Hourly.Error.ArchiveNeverWritten) ] ] ,COP(@78ebd086@[4],@90f69b4d@.Archive.Fetch.Hourly.Default.ClosingTimestamp,1) ,COP(@78ebd086@[6],@90f69b4d@.Archive.Fetch.Hourly.Default.CumulativeActiveStreams,1) ,COP(@78ebd086@[7],@6765098e@,1) [MVM(@6765098e@,16#0000000F,@a2e06d14@) ADD(@a2e06d14@,1,@90f69b4d@.Archive.Fetch.Hourly.Default.CurrentActiveStream) ,MVM(@6765098e@,16#0000FF00,@207884c7@) DIV(@207884c7@,256,@207884c7@) COP(@207884c7@,@90f69b4d@.Archive.Fetch.Hourly.Default.MeterStatus,1) ] ,COP(@78ebd086@[8],@90f69b4d@.Archive.Fetch.Hourly.Default.FlowingPeriod,48) ,COP(@78ebd086@[4],@90f69b4d@.Archive.Fetch.Hourly.Raw[0],100) ] ,XIC(@90f69b4d@.Archive.Fetch.Daily.Trigger) [OTU(@90f69b4d@.Archive.Fetch.Daily.Trigger) ,[[XIC(@78ebd086@[105].0) OTL(@90f69b4d@.Archive.Fetch.Daily.Error.ArchiveSelectionInvalid) ,XIO(@78ebd086@[105].0) OTU(@90f69b4d@.Archive.Fetch.Daily.Error.ArchiveSelectionInvalid) ] ,[XIC(@78ebd086@[105].1) OTL(@90f69b4d@.Archive.Fetch.Daily.Error.AgeOutsideSize) ,XIO(@78ebd086@[105].1) OTU(@90f69b4d@.Archive.Fetch.Daily.Error.AgeOutsideSize) ] ,[XIC(@78ebd086@[105].2) OTL(@90f69b4d@.Archive.Fetch.Daily.Error.ArchiveNeverWritten) ,XIO(@78ebd086@[105].2) OTU(@90f69b4d@.Archive.Fetch.Daily.Error.ArchiveNeverWritten) ] ] ,COP(@78ebd086@[106],@90f69b4d@.Archive.Fetch.Daily.Default.ClosingTimestamp,1) ,COP(@78ebd086@[108],@90f69b4d@.Archive.Fetch.Daily.Default.CumulativeActiveStreams,1) ,COP(@78ebd086@[109],@6765098e@,1) [MVM(@6765098e@,16#0000000F,@a2e06d14@) ADD(@a2e06d14@,1,@90f69b4d@.Archive.Fetch.Daily.Default.CurrentActiveStream) ,MVM(@6765098e@,16#0000FF00,@207884c7@) DIV(@207884c7@,256,@207884c7@) COP(@207884c7@,@90f69b4d@.Archive.Fetch.Daily.Default.MeterStatus,1) ] ,COP(@78ebd086@[110],@90f69b4d@.Archive.Fetch.Daily.Default.FlowingPeriod,48) ,COP(@78ebd086@[106],@90f69b4d@.Archive.Fetch.Daily.Raw[0],100) ] ,MVM(16#0000,@3ca1aa1f@,@99473fd2@.Util.Block.NonInterruptPending.Archive) MVM(16#FFFF,@3ca1aa1f@,@99473fd2@.Util.Block.NonInterruptComplete.Archive) OTU(@99473fd2@.Util.Block.NonInterruptPending.Now) ];
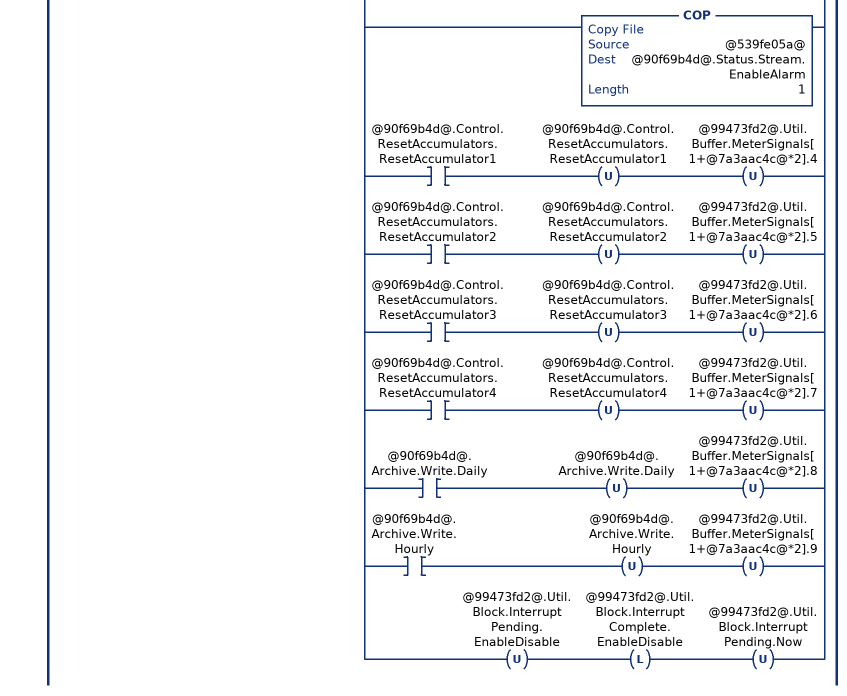
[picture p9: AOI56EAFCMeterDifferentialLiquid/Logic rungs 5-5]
   // Meter status and stream status.
   // Remove trigger and pending flags.
   5: XIC(@bc637796@)EQU(@78ebd086@[0],7000)[[MVM(@78ebd086@[3],@3ca1aa1f@,@449238e1@) ,[NEQ(@449238e1@,0) OTL(@90f69b4d@.Status.Meter.Enabled) ,EQU(@449238e1@,0) OTU(@90f69b4d@.Status.Meter.Enabled) ] ,OTU(@90f69b4d@.Control.Meter.Enable) MVM(16#0000,@3ca1aa1f@,@99473fd2@.Util.Buffer.MeterEnableDisable[1]) ,OTU(@90f69b4d@.Control.Meter.Disable) MVM(16#0000,@3ca1aa1f@,@99473fd2@.Util.Buffer.MeterEnableDisable[3]) ] ,[XIC(@90f69b4d@.Control.Stream.EnableSelected) [COP(@78ebd086@[7+@7a3aac4c@*3],@90f69b4d@.Status.Stream.Enabled,1) ,COP(@78ebd086@[8+@7a3aac4c@*3],@90f69b4d@.Status.Stream.Configured,1) ,OTU(@90f69b4d@.Control.Stream.EnableSelected) OTU(@90f69b4d@.Control.Stream.DisableSelected) ] ,XIC(@90f69b4d@.Control.Stream.DisableSelected) [COP(@78ebd086@[55+@7a3aac4c@*3],@90f69b4d@.Status.Stream.Enabled,1) ,COP(@78ebd086@[56+@7a3aac4c@*3],@90f69b4d@.Status.Stream.Configured,1) ,OTU(@90f69b4d@.Control.Stream.EnableSelected) OTU(@90f69b4d@.Control.Stream.DisableSelected) ] ] ,[OTU(@90f69b4d@.Control.Stream.SetSelectedToActive) ,COP(@78ebd086@[103+@7a3aac4c@*2],@25207d76@,1) ,[XIC(@25207d76@.8) OTL(@539fe05a@.0) ,XIO(@25207d76@.8) OTU(@539fe05a@.0) ] ,[XIC(@25207d76@.9) OTL(@539fe05a@.1) ,XIO(@25207d76@.9) OTU(@539fe05a@.1) ] ,[XIC(@25207d76@.10) OTL(@539fe05a@.2) ,XIO(@25207d76@.10) OTU(@539fe05a@.2) ] ,[XIC(@25207d76@.11) OTL(@539fe05a@.3) ,XIO(@25207d76@.11) OTU(@539fe05a@.3) ] ,MVM(@25207d76@,16#000F,@5babdfcf@) ADD(@5babdfcf@,1,@90f69b4d@.Status.Stream.Active) ,COP(@539fe05a@,@90f69b4d@.Status.Stream.EnableAlarm,1) ] ,[XIC(@90f69b4d@.Control.ResetAccumulators.ResetAccumulator1) OTU(@90f69b4d@.Control.ResetAccumulators.ResetAccumulator1) OTU(@99473fd2@.Util.Buffer.MeterSignals[1+@7a3aac4c@*2].4) ,XIC(@90f69b4d@.Control.ResetAccumulators.ResetAccumulator2) OTU(@90f69b4d@.Control.ResetAccumulators.ResetAccumulator2) OTU(@99473fd2@.Util.Buffer.MeterSignals[1+@7a3aac4c@*2].5) ,XIC(@90f69b4d@.Control.ResetAccumulators.ResetAccumulator3) OTU(@90f69b4d@.Control.ResetAccumulators.ResetAccumulator3) OTU(@99473fd2@.Util.Buffer.MeterSignals[1+@7a3aac4c@*2].6) ,XIC(@90f69b4d@.Control.ResetAccumulators.ResetAccumulator4) OTU(@90f69b4d@.Control.ResetAccumulators.ResetAccumulator4) OTU(@99473fd2@.Util.Buffer.MeterSignals[1+@7a3aac4c@*2].7) ,XIC(@90f69b4d@.Archive.Write.Daily) OTU(@90f69b4d@.Archive.Write.Daily) OTU(@99473fd2@.Util.Buffer.MeterSignals[1+@7a3aac4c@*2].8) ,XIC(@90f69b4d@.Archive.Write.Hourly) OTU(@90f69b4d@.Archive.Write.Hourly) OTU(@99473fd2@.Util.Buffer.MeterSignals[1+@7a3aac4c@*2].9) ] ,OTU(@99473fd2@.Util.Block.InterruptPending.EnableDisable) OTL(@99473fd2@.Util.Block.InterruptComplete.EnableDisable) OTU(@99473fd2@.Util.Block.InterruptPending.Now) ];
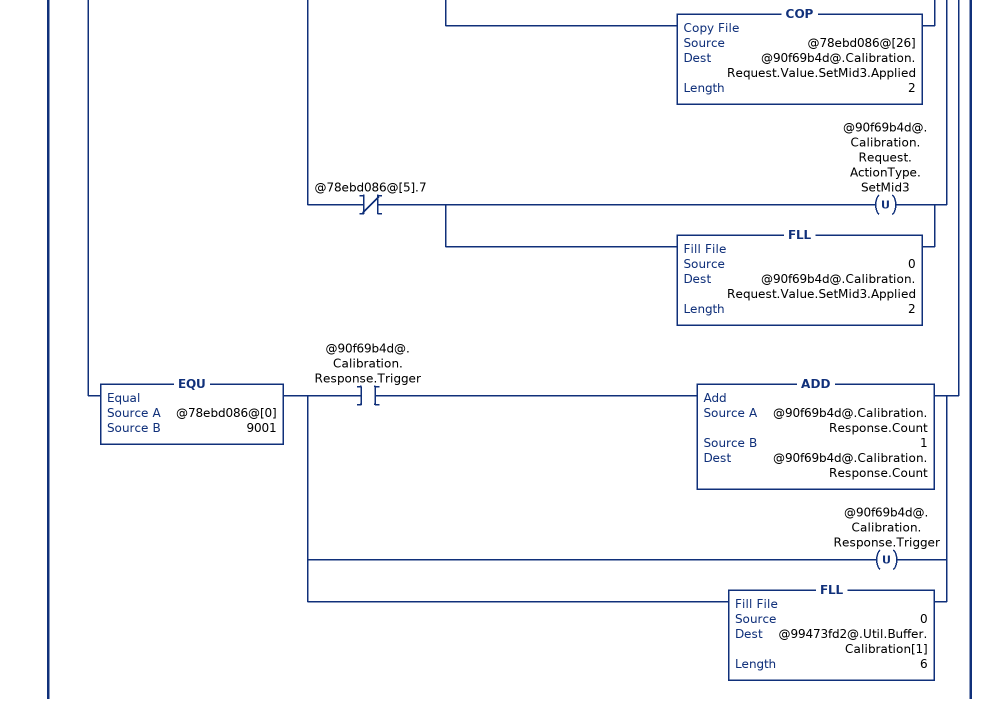
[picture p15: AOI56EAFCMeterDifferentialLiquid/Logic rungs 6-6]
   // Meter transmitter calibration.
   6: XIC(@bc637796@)[EQU(@78ebd086@[0],9000) ,EQU(@78ebd086@[0],9001) ][MVM(@78ebd086@[3],16#0F00,@d70169b1@) ,DIV(@d70169b1@,16#100,@d70169b1@) ]EQU(@d70169b1@,@7a3aac4c@)XIO(@78ebd086@[3].14)[EQU(@78ebd086@[0],9000) [XIO(@9ee3b510@) ADD(@90f69b4d@.Calibration.Request.Count,1,@90f69b4d@.Calibration.Request.Count) ,OTL(@9ee3b510@) [COP(@78ebd086@[3],@2350f06a@,1) ,MVM(@2350f06a@,16#000F,@100b5a53@) ] ,[EQU(@100b5a53@,0) [OTL(@90f69b4d@.Calibration.Request.ProcessVariable.DifferentialPressure) ,OTU(@90f69b4d@.Calibration.Request.ProcessVariable.Temperature) ,OTU(@90f69b4d@.Calibration.Request.ProcessVariable.Pressure) ,OTU(@90f69b4d@.Calibration.Request.ProcessVariable.Density) ,OTU(@90f69b4d@.Calibration.Request.ProcessVariable.WaterContent) ] ,EQU(@100b5a53@,1) [OTL(@90f69b4d@.Calibration.Request.ProcessVariable.Temperature) ,OTU(@90f69b4d@.Calibration.Request.ProcessVariable.DifferentialPressure) ,OTU(@90f69b4d@.Calibration.Request.ProcessVariable.Pressure) ,OTU(@90f69b4d@.Calibration.Request.ProcessVariable.Density) ,OTU(@90f69b4d@.Calibration.Request.ProcessVariable.WaterContent) ] ,EQU(@100b5a53@,2) [OTL(@90f69b4d@.Calibration.Request.ProcessVariable.Pressure) ,OTU(@90f69b4d@.Calibration.Request.ProcessVariable.DifferentialPressure) ,OTU(@90f69b4d@.Calibration.Request.ProcessVariable.Temperature) ,OTU(@90f69b4d@.Calibration.Request.ProcessVariable.Density) ,OTU(@90f69b4d@.Calibration.Request.ProcessVariable.WaterContent) ] ,EQU(@100b5a53@,3) [OTL(@90f69b4d@.Calibration.Request.ProcessVariable.Density) ,OTU(@90f69b4d@.Calibration.Request.ProcessVariable.DifferentialPressure) ,OTU(@90f69b4d@.Calibration.Request.ProcessVariable.Temperature) ,OTU(@90f69b4d@.Calibration.Request.ProcessVariable.Pressure) ,OTU(@90f69b4d@.Calibration.Request.ProcessVariable.WaterContent) ] ,EQU(@100b5a53@,4) [OTL(@90f69b4d@.Calibration.Request.ProcessVariable.WaterContent) ,OTU(@90f69b4d@.Calibration.Request.ProcessVariable.DifferentialPressure) ,OTU(@90f69b4d@.Calibration.Request.ProcessVariable.Temperature) ,OTU(@90f69b4d@.Calibration.Request.ProcessVariable.Pressure) ,OTU(@90f69b4d@.Calibration.Request.ProcessVariable.Density) ] ] ,[[XIC(@78ebd086@[5].2) [OTL(@90f69b4d@.Calibration.Request.ActionType.ZeroShift) ,COP(@78ebd086@[6],@90f69b4d@.Calibration.Request.Value.ZeroShift.Applied,2) ] ,XIO(@78ebd086@[5].2) [OTU(@90f69b4d@.Calibration.Request.ActionType.ZeroShift) ,FLL(0,@90f69b4d@.Calibration.Request.Value.ZeroShift.Applied,2) ] ] ,[XIC(@78ebd086@[5].3) [OTL(@90f69b4d@.Calibration.Request.ActionType.SetZero) ,COP(@78ebd086@[10],@90f69b4d@.Calibration.Request.Value.SetZero.Applied,2) ] ,XIO(@78ebd086@[5].3) [OTU(@90f69b4d@.Calibration.Request.ActionType.SetZero) ,FLL(0,@90f69b4d@.Calibration.Request.Value.SetZero.Applied,2) ] ] ,[XIC(@78ebd086@[5].4) [OTL(@90f69b4d@.Calibration.Request.ActionType.SetSpan) ,COP(@78ebd086@[14],@90f69b4d@.Calibration.Request.Value.SetSpan.Applied,2) ] ,XIO(@78ebd086@[5].4) [OTU(@90f69b4d@.Calibration.Request.ActionType.SetSpan) ,FLL(0,@90f69b4d@.Calibration.Request.Value.SetSpan.Applied,2) ] ] ,[XIC(@78ebd086@[5].5) [OTL(@90f69b4d@.Calibration.Request.ActionType.SetMid1) ,COP(@78ebd086@[18],@90f69b4d@.Calibration.Request.Value.SetMid1.Applied,2) ] ,XIO(@78ebd086@[5].5) [OTU(@90f69b4d@.Calibration.Request.ActionType.SetMid1) ,FLL(0,@90f69b4d@.Calibration.Request.Value.SetMid1.Applied,2) ] ] ,[XIC(@78ebd086@[5].6) [OTL(@90f69b4d@.Calibration.Request.ActionType.SetMid2) ,COP(@78ebd086@[22],@90f69b4d@.Calibration.Request.Value.SetMid2.Applied,2) ] ,XIO(@78ebd086@[5].6) [OTU(@90f69b4d@.Calibration.Request.ActionType.SetMid2) ,FLL(0,@90f69b4d@.Calibration.Request.Value.SetMid2.Applied,2) ] ] ,[XIC(@78ebd086@[5].7) [OTL(@90f69b4d@.Calibration.Request.ActionType.SetMid3) ,COP(@78ebd086@[26],@90f69b4d@.Calibration.Request.Value.SetMid3.Applied,2) ] ,XIO(@78ebd086@[5].7) [OTU(@90f69b4d@.Calibration.Request.ActionType.SetMid3) ,FLL(0,@90f69b4d@.Calibration.Request.Value.SetMid3.Applied,2) ] ] ] ] ,EQU(@78ebd086@[0],9001) [XIC(@90f69b4d@.Calibration.Response.Trigger) ADD(@90f69b4d@.Calibration.Response.Count,1,@90f69b4d@.Calibration.Response.Count) ,OTU(@90f69b4d@.Calibration.Response.Trigger) ,FLL(0,@99473fd2@.Util.Buffer.Calibration[1],6) ] ];
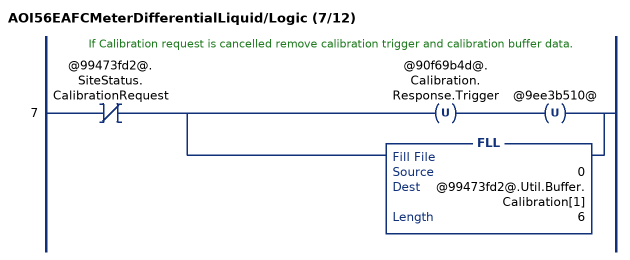
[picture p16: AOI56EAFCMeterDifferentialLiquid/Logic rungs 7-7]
   // If Calibration request is cancelled remove calibration trigger and calibration buffer data.
   7: XIO(@99473fd2@.SiteStatus.CalibrationRequest)[OTU(@90f69b4d@.Calibration.Response.Trigger) OTU(@9ee3b510@) ,FLL(0,@99473fd2@.Util.Buffer.Calibration[1],6) ];
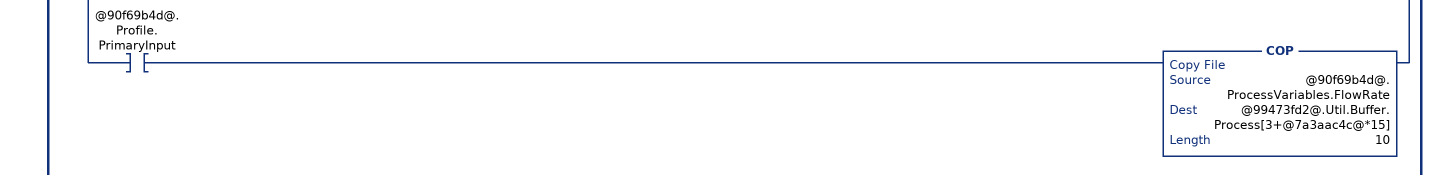
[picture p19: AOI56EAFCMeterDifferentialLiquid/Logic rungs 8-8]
   // Process variables and process alarms to send to module.
   8: XIC(@a002d86f@)[ADD(16#A000,@989351bc@,@73ebb0c9@) COP(@73ebb0c9@,@99473fd2@.Util.Buffer.Process[@7a3aac4c@*15],1) ,[XIO(@90f69b4d@.Profile.PrimaryInput) XIC(@90f69b4d@.Alarm.Control.DifferentialPressure.SetAutoClearStaleData) OTU(@90f69b4d@.Alarm.Control.DifferentialPressure.StaleData) ,XIC(@90f69b4d@.Profile.PrimaryInput) XIC(@90f69b4d@.Alarm.Control.FlowRate.SetAutoClearStaleData) OTU(@90f69b4d@.Alarm.Control.FlowRate.StaleData) ,XIO(@90f69b4d@.Profile.PrimaryInput) COP(@90f69b4d@.Alarm.Control.DifferentialPressure,@99473fd2@.Util.Buffer.Process[1+@7a3aac4c@*15],1) OTL(@90f69b4d@.Alarm.Control.DifferentialPressure.StaleData) ,XIC(@90f69b4d@.Profile.PrimaryInput) COP(@90f69b4d@.Alarm.Control.FlowRate,@99473fd2@.Util.Buffer.Process[1+@7a3aac4c@*15],1) OTL(@90f69b4d@.Alarm.Control.FlowRate.StaleData) ] ,[XIC(@90f69b4d@.Alarm.Control.Temperature.SetAutoClearStaleData) OTU(@90f69b4d@.Alarm.Control.Temperature.StaleData) ,COP(@90f69b4d@.Alarm.Control.Temperature,@0a7565e2@,1) MUL(@0a7565e2@,16,@447f2ec8@) MVM(@447f2ec8@,16#00F0,@99473fd2@.Util.Buffer.Process[1+@7a3aac4c@*15]) OTL(@90f69b4d@.Alarm.Control.Temperature.StaleData) ] ,[XIC(@90f69b4d@.Alarm.Control.Pressure.SetAutoClearStaleData) OTU(@90f69b4d@.Alarm.Control.Pressure.StaleData) ,COP(@90f69b4d@.Alarm.Control.Pressure,@0a7565e2@,1) MUL(@0a7565e2@,256,@447f2ec8@) MVM(@447f2ec8@,16#0F00,@99473fd2@.Util.Buffer.Process[1+@7a3aac4c@*15]) OTL(@90f69b4d@.Alarm.Control.Pressure.StaleData) ] ,[XIC(@90f69b4d@.Alarm.Control.Density.SetAutoClearStaleData) OTU(@90f69b4d@.Alarm.Control.Density.StaleData) ,COP(@90f69b4d@.Alarm.Control.Density,@0a7565e2@,1) COP(@99473fd2@.Util.Buffer.Process[1+@7a3aac4c@*15],@acc7602b@,1) MUL(@0a7565e2@,4096,@447f2ec8@) MVM(@447f2ec8@,16#F000,@acc7602b@) COP(@acc7602b@,@99473fd2@.Util.Buffer.Process[1+@7a3aac4c@*15],1) OTL(@90f69b4d@.Alarm.Control.Density.StaleData) ] ,[XIC(@90f69b4d@.Alarm.Control.WaterPercent.SetAutoClearStaleData) OTU(@90f69b4d@.Alarm.Control.WaterPercent.StaleData) ,COP(@90f69b4d@.Alarm.Control.WaterPercent,@99473fd2@.Util.Buffer.Process[2+@7a3aac4c@*15],2) OTL(@90f69b4d@.Alarm.Control.WaterPercent.StaleData) ] ,XIO(@90f69b4d@.Profile.PrimaryInput) [COP(@90f69b4d@.ProcessVariables.DifferentialPressure,@99473fd2@.Util.Buffer.Process[3+@7a3aac4c@*15],2) ,COP(@90f69b4d@.ProcessVariables.Temperature,@99473fd2@.Util.Buffer.Process[3+2+@7a3aac4c@*15],8) ] ,XIC(@90f69b4d@.Profile.PrimaryInput) COP(@90f69b4d@.ProcessVariables.FlowRate,@99473fd2@.Util.Buffer.Process[3+@7a3aac4c@*15],10) ];
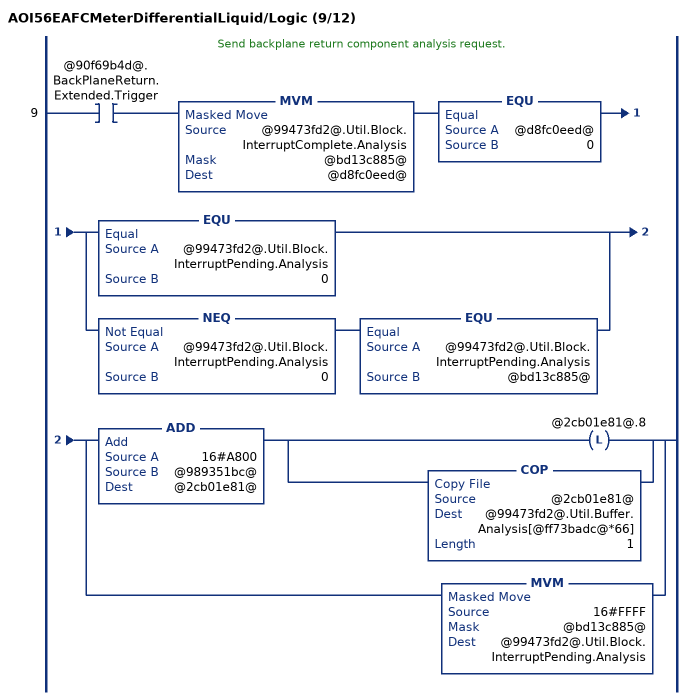
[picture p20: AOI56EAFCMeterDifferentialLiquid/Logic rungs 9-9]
   // Send backplane return component analysis request.
   9: XIC(@90f69b4d@.BackPlaneReturn.Extended.Trigger)MVM(@99473fd2@.Util.Block.InterruptComplete.Analysis,@bd13c885@,@d8fc0eed@)EQU(@d8fc0eed@,0)[EQU(@99473fd2@.Util.Block.InterruptPending.Analysis,0) ,NEQ(@99473fd2@.Util.Block.InterruptPending.Analysis,0) EQU(@99473fd2@.Util.Block.InterruptPending.Analysis,@bd13c885@) ][ADD(16#A800,@989351bc@,@2cb01e81@) [OTL(@2cb01e81@.8) ,COP(@2cb01e81@,@99473fd2@.Util.Buffer.Analysis[@ff73badc@*66],1) ] ,MVM(16#FFFF,@bd13c885@,@99473fd2@.Util.Block.InterruptPending.Analysis) ];
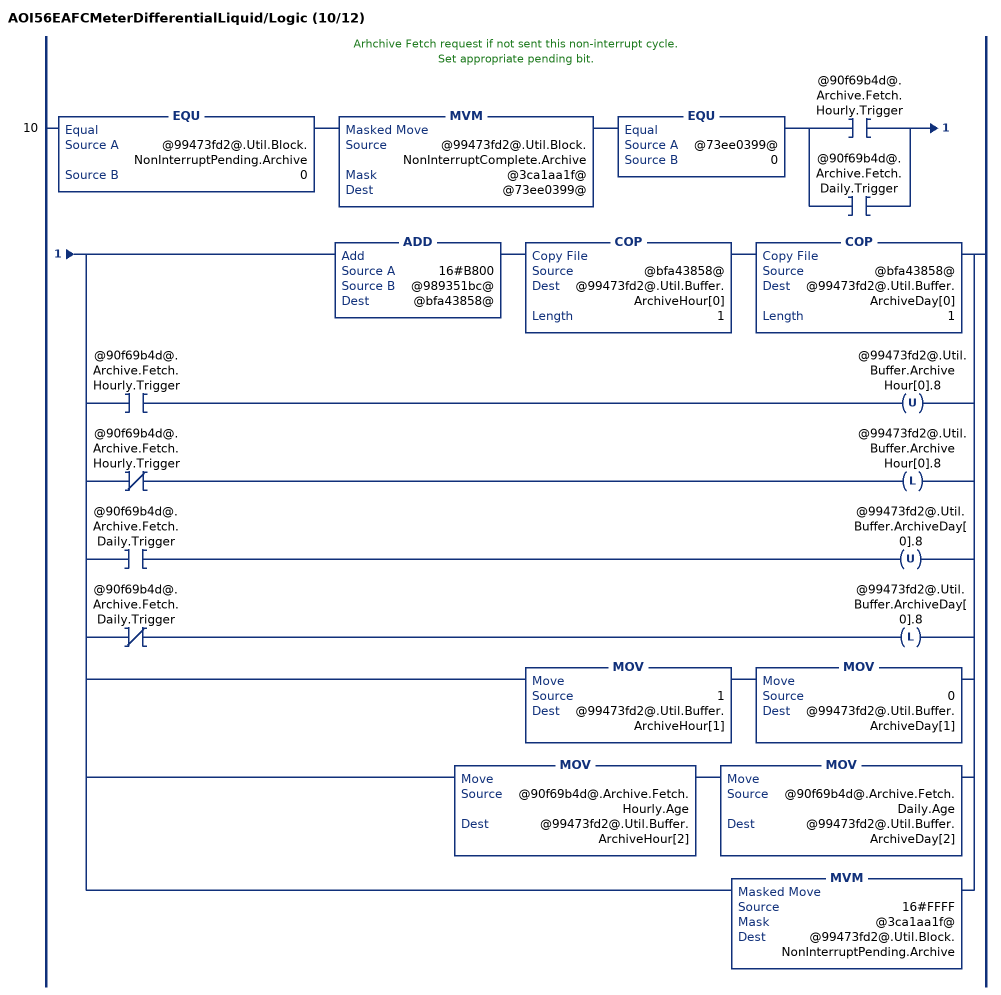
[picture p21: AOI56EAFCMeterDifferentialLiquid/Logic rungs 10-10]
   // Arhchive Fetch request if not sent this non-interrupt cycle.
   // Set appropriate pending bit.
   10: EQU(@99473fd2@.Util.Block.NonInterruptPending.Archive,0)MVM(@99473fd2@.Util.Block.NonInterruptComplete.Archive,@3ca1aa1f@,@73ee0399@)EQU(@73ee0399@,0)[XIC(@90f69b4d@.Archive.Fetch.Hourly.Trigger) ,XIC(@90f69b4d@.Archive.Fetch.Daily.Trigger) ][ADD(16#B800,@989351bc@,@bfa43858@) COP(@bfa43858@,@99473fd2@.Util.Buffer.ArchiveHour[0],1) COP(@bfa43858@,@99473fd2@.Util.Buffer.ArchiveDay[0],1) ,[XIC(@90f69b4d@.Archive.Fetch.Hourly.Trigger) OTU(@99473fd2@.Util.Buffer.ArchiveHour[0].8) ,XIO(@90f69b4d@.Archive.Fetch.Hourly.Trigger) OTL(@99473fd2@.Util.Buffer.ArchiveHour[0].8) ] ,[XIC(@90f69b4d@.Archive.Fetch.Daily.Trigger) OTU(@99473fd2@.Util.Buffer.ArchiveDay[0].8) ,XIO(@90f69b4d@.Archive.Fetch.Daily.Trigger) OTL(@99473fd2@.Util.Buffer.ArchiveDay[0].8) ] ,MOV(1,@99473fd2@.Util.Buffer.ArchiveHour[1]) MOV(0,@99473fd2@.Util.Buffer.ArchiveDay[1]) ,MOV(@90f69b4d@.Archive.Fetch.Hourly.Age,@99473fd2@.Util.Buffer.ArchiveHour[2]) MOV(@90f69b4d@.Archive.Fetch.Daily.Age,@99473fd2@.Util.Buffer.ArchiveDay[2]) ,MVM(16#FFFF,@3ca1aa1f@,@99473fd2@.Util.Block.NonInterruptPending.Archive) ];
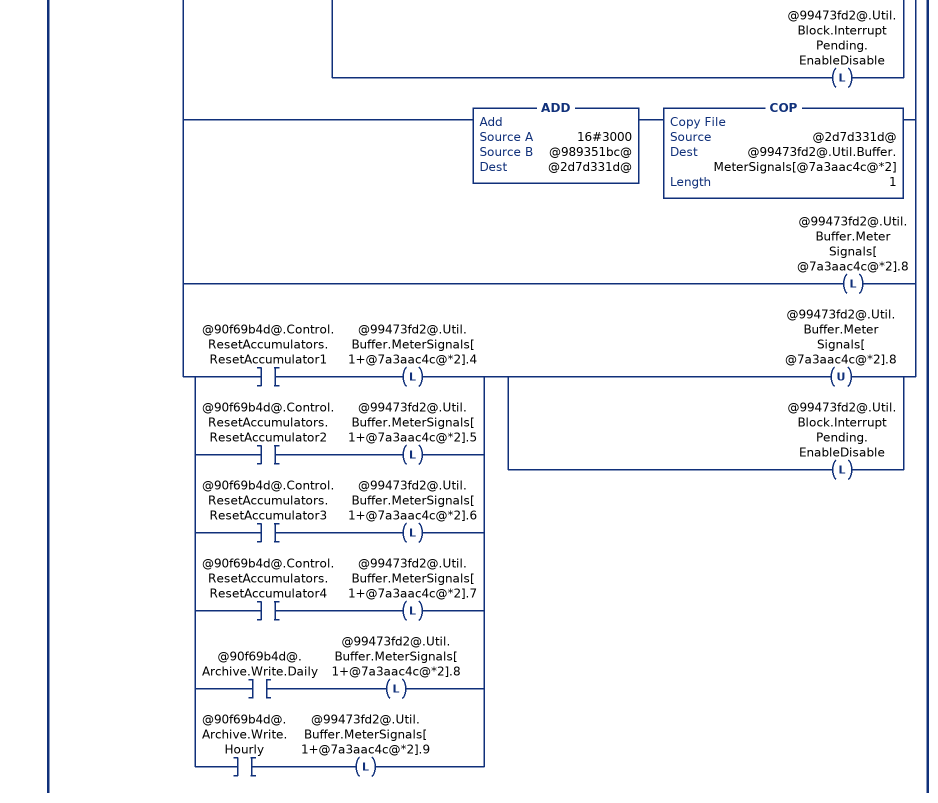
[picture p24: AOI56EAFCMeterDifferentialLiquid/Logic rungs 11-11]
   // Meter Enable.
   // Meter Disable.
   // Stream Select.
   // Stream Enable.
   // Stream Disable.
   // Set pending bit if not set this interrupt cycle.
   11: XIO(@99473fd2@.Util.Block.InterruptComplete.EnableDisable)[LIM(1,@90f69b4d@.Control.Stream.Selected,16) CPT(@89d45884@,2**(@90f69b4d@.Control.Stream.Selected-1)) ,[XIC(@90f69b4d@.Control.Meter.Enable) MVM(16#FFFF,@3ca1aa1f@,@99473fd2@.Util.Buffer.MeterEnableDisable[1]) MVM(16#0000,@3ca1aa1f@,@99473fd2@.Util.Buffer.MeterEnableDisable[3]) ,XIC(@90f69b4d@.Control.Meter.Disable) MVM(16#FFFF,@3ca1aa1f@,@99473fd2@.Util.Buffer.MeterEnableDisable[3]) MVM(16#0000,@3ca1aa1f@,@99473fd2@.Util.Buffer.MeterEnableDisable[1]) ] OTL(@99473fd2@.Util.Block.InterruptPending.EnableDisable) ,[ADD(16#CC00,@989351bc@,@47fbaeb5@) COP(@47fbaeb5@,@99473fd2@.Util.Buffer.StreamEnable[@7a3aac4c@*3],1) ,XIO(@90f69b4d@.Control.Stream.EnableSelected) OTL(@99473fd2@.Util.Buffer.StreamEnable[@7a3aac4c@*3].8) ,XIC(@90f69b4d@.Control.Stream.EnableSelected) [OTU(@99473fd2@.Util.Buffer.StreamEnable[@7a3aac4c@*3].8) ,COP(@89d45884@,@99473fd2@.Util.Buffer.StreamEnable[1+@7a3aac4c@*3],1) ,OTL(@99473fd2@.Util.Block.InterruptPending.EnableDisable) ] ] ,[ADD(16#C800,@989351bc@,@8034a877@) COP(@8034a877@,@99473fd2@.Util.Buffer.StreamDisable[@7a3aac4c@*3],1) ,XIO(@90f69b4d@.Control.Stream.DisableSelected) OTL(@99473fd2@.Util.Buffer.StreamDisable[@7a3aac4c@*3].8) ,XIC(@90f69b4d@.Control.Stream.DisableSelected) [OTU(@99473fd2@.Util.Buffer.StreamDisable[@7a3aac4c@*3].8) ,COP(@89d45884@,@99473fd2@.Util.Buffer.StreamDisable[1+@7a3aac4c@*3],1) ,OTL(@99473fd2@.Util.Block.InterruptPending.EnableDisable) ] ] ,[ADD(16#3C00,@989351bc@,@5da28580@) COP(@5da28580@,@99473fd2@.Util.Buffer.StreamSelect[@7a3aac4c@*2],1) ,XIO(@90f69b4d@.Control.Stream.SetSelectedToActive) OTL(@99473fd2@.Util.Buffer.StreamSelect[@7a3aac4c@*2].8) ,XIC(@90f69b4d@.Control.Stream.SetSelectedToActive) [OTU(@99473fd2@.Util.Buffer.StreamSelect[@7a3aac4c@*2].8) ,MOV(@90f69b4d@.Control.Stream.Selected,@99473fd2@.Util.Buffer.StreamSelect[1+@7a3aac4c@*2]) ,OTL(@99473fd2@.Util.Block.InterruptPending.EnableDisable) ] ] ,[ADD(16#3000,@989351bc@,@2d7d331d@) COP(@2d7d331d@,@99473fd2@.Util.Buffer.MeterSignals[@7a3aac4c@*2],1) ,OTL(@99473fd2@.Util.Buffer.MeterSignals[@7a3aac4c@*2].8) ,[XIC(@90f69b4d@.Control.ResetAccumulators.ResetAccumulator1) OTL(@99473fd2@.Util.Buffer.MeterSignals[1+@7a3aac4c@*2].4) ,XIC(@90f69b4d@.Control.ResetAccumulators.ResetAccumulator2) OTL(@99473fd2@.Util.Buffer.MeterSignals[1+@7a3aac4c@*2].5) ,XIC(@90f69b4d@.Control.ResetAccumulators.ResetAccumulator3) OTL(@99473fd2@.Util.Buffer.MeterSignals[1+@7a3aac4c@*2].6) ,XIC(@90f69b4d@.Control.ResetAccumulators.ResetAccumulator4) OTL(@99473fd2@.Util.Buffer.MeterSignals[1+@7a3aac4c@*2].7) ,XIC(@90f69b4d@.Archive.Write.Daily) OTL(@99473fd2@.Util.Buffer.MeterSignals[1+@7a3aac4c@*2].8) ,XIC(@90f69b4d@.Archive.Write.Hourly) OTL(@99473fd2@.Util.Buffer.MeterSignals[1+@7a3aac4c@*2].9) ] [OTU(@99473fd2@.Util.Buffer.MeterSignals[@7a3aac4c@*2].8) ,OTL(@99473fd2@.Util.Block.InterruptPending.EnableDisable) ] ] ];
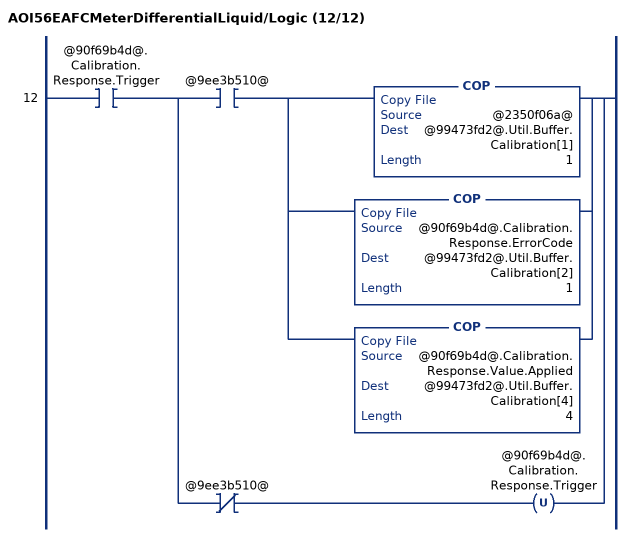
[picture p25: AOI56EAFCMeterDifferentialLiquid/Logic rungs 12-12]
   12: XIC(@90f69b4d@.Calibration.Response.Trigger)[XIC(@9ee3b510@) [COP(@2350f06a@,@99473fd2@.Util.Buffer.Calibration[1],1) ,COP(@90f69b4d@.Calibration.Response.ErrorCode,@99473fd2@.Util.Buffer.Calibration[2],1) ,COP(@90f69b4d@.Calibration.Response.Value.Applied,@99473fd2@.Util.Buffer.Calibration[4],4) ] ,XIO(@9ee3b510@) OTU(@90f69b4d@.Calibration.Response.Trigger) ];
END_ROUTINE

ROUTINE Prescan   (* ladder *)
END_ROUTINE
END_ADD_ON_INSTRUCTION

VAR_GLOBAL   (* controller tags *)
   AOI56EAFCMeter02DifferentialLiquid : AOI56EAFCMeterDifferentialLiquid;
   AFC : AFCEModuleDef;
   Local:1:I : AB:1756_MODULE_INT_500Bytes:I:0;
   AFCMeter02DifferentialLiquid : AFCEMeterDifferentialLiquid;
END_VAR

PROGRAM MainProgram

ROUTINE MainRoutine   (* ladder *)
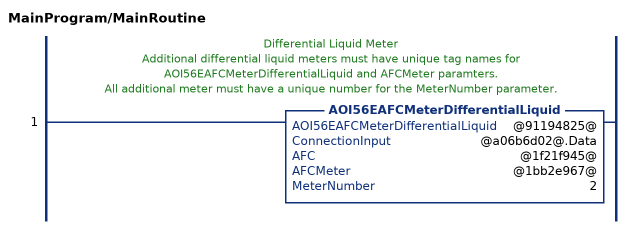
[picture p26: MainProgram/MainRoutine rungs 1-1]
   // Differential Liquid Meter
   // Additional differential liquid meters must have unique tag names for AOI56EAFCMeterDifferentialLiquid and AFCMeter paramters.
   // All additional meter must have a unique number for the MeterNumber parameter.
   1: AOI56EAFCMeterDifferentialLiquid(@91194825@,@a06b6d02@.Data,@1f21f945@,@1bb2e967@,2);
END_ROUTINE
END_PROGRAM
